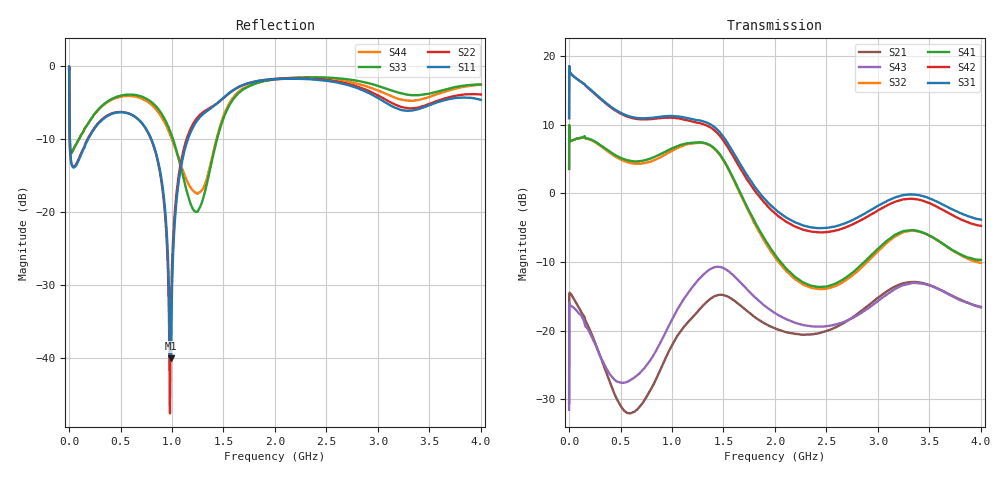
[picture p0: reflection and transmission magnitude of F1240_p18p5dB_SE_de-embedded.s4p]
! Integrated Device Technology
! Corporate Headquarters
! 6024 Silver Creek Valley Road
! San Jose, CA 95138  USA
! Phone:  1-408-284-8200
! Toll Free:  1-800-223-1366
! Webpage:  http://www.idt.com/
! Timing and RF Division
! 515 Groton Road, Suite 102
! Westford, MA 01886-6024
! Device:  F1240
! Description: Dual Intermediate Frequency Digital Variable Gain Amplifier
! Frequency:  10.0 -  500.00 MHz
! Package:  5x5 mm QFN Plastic Package: 32 pin
! Ports:  8 RF, 20 DC
!  Pin  1  = GA3 / Data  Pin 17  = RF OUT_B+
!  Pin  2  = GA4 / CLK  Pin 18  = RF OUT_B-
!  Pin  3  = GA5  Pin 19  = STBY_B
!  Pin  4  = VMODE  Pin 20  = Ground
!  Pin  5  = No Connect  Pin 21  = Ground
!  Pin  6  = GB5  Pin 22  = STB_A
!  Pin  7  = GB4  Pin 23  = RF OUT_A-  = Port 4
!  Pin  8  = GB3  Pin 24  = RF OUT_A+  = Port 3
!  Pin  9  = GB2  Pin 25  = GA0
!  Pin 10  = GB1  Pin 26  = ISET_A
!  Pin 11  = RF IN_B+  Pin 27  = VCC
!  Pin 12  = RF IN_B-  Pin 28  = Ground
!  Pin 13  = Ground  Pin 29  = RF IN_A-  = Port 2
!  Pin 14  = VCC  Pin 30  = RF IN_A+  = Port 1
!  Pin 15  = ISET_B  Pin 31  = GA1
!  Pin 16  = GB0  Pin 32  = GA2 / CSb
! Gain  = +19.5 dB
! State  = 1
! Voltage  = +5.00 V
! Current  = 85.292 mA (one channel only)
! Temperture  =  +25 C
! Test Date  =  2017-10-18
! Board  =  EB4031
! Data:  The device was measured on a custom evaluation board which has
!  individual transmission lines to the RF pins.  Data was collected
!  using a calibrated network analyzer.  The evaluation board was
!  de-embedded using Automatic Fixture Removal.
!  The reference plane is the edge of the package pin.
!  Only Channel A was measured.
!  This data is in single-ended operation.  If your needs are balanced
!  or differential S-parameters then this file needs to be used a
!  linear simulator.
! File Date:  2017-11-10  MJV
! Note:
!  Integrated Device Technology supplies this data as a sample of measured
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# Hz S dB R 100
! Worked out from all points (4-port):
!   410 points, 500 kHz to 4 GHz, reference 100 ohm
!   strongest paths, dB at 500 kHz, 930 MHz, 1.96 GHz, 2.98 GHz, 4 GHz:
!     S31: 11.0, 11.2, -1.8, -2.0, -3.8
!     S42: 10.9, 11.0, -2.4, -2.7, -4.7
!     S41: 3.5, 6.0, -8.1, -8.4, -9.7
!     S32: 3.5, 5.6, -8.5, -8.8, -10.1
!     S43: -31.5, -20.5, -17.1, -15.9, -16.5
!     S21: -30.6, -24.3, -19.4, -15.5, -16.6
!   lowest |S11| = -40.0 dB at 990 MHz (marker M1), VSWR 1.02, Z = 101 - j1.89 ohm
!   |S11| at or under -10 dB: 7.315 MHz to 183.5 MHz (176.2 MHz wide, 185 % of centre); 800.1 MHz to 1.153 GHz (353.1 MHz wide, 36.2 % of centre)
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500000  -0.28 -6.7  -30.39 27.2  -27.54 71.4  -64.34 71.3
        -30.57 26.5  -0.27 -6.6  -63.97 65.9  -27.55 72.5
        10.95 -105.6  3.54 72.6  -0.39 0.6  -31.58 -174.7
        3.54 73.6  10.93 -104.4  -31.54 -174.8  -0.40 3.0
3500000  -6.39 -49.9  -14.55 14.8  -21.30 7.1  -38.64 42.3
         -14.56 14.7  -6.36 -50.0  -38.60 42.2  -21.31 7.2
         18.14 -171.8  8.30 -1.1  -6.05 -44.7  -16.10 25.3
         8.29 -1.1  18.13 -171.6  -16.07 25.2  -6.10 -44.5
2.1e8  -9.33 -110.6  -20.17 -111.1  -24.08 -52.3  -33.44 7.8
       -20.20 -109.9  -9.19 -112.4  -33.46 7.8  -24.10 -52.2
       15.10 106.5  7.76 -61.4  -7.26 -79.5  -20.09 -118.6
       7.85 -61.3  15.03 105.6  -20.62 -117.2  -7.29 -78.8
5.6e8  -6.38 -172.2  -31.15 93.4  -25.65 -107.5  -27.51 -61.3
       -31.98 91.5  -6.35 -173.6  -27.68 -60.1  -25.82 -107.8
       11.33 19.8  4.55 -146.2  -3.87 -151.4  -26.39 91.3
       4.83 -147.1  11.20 18.7  -27.50 68.5  -4.04 -150.8
9.9e8  -39.99 -70.0  -20.56 -32.2  -22.54 164.1  -22.61 -162.8
       -22.43 -32.5  -32.93 -58.3  -22.97 -158.5  -22.98 163.6
       11.26 -83.9  6.10 120.9  -9.19 146.8  -17.37 -11.3
       6.47 115.9  11.01 -85.7  -18.69 -34.2  -9.63 153.2
1.5e9  -4.28 -138.4  -14.87 166.6  -29.55 43.3  -24.07 69.5
       -14.84 171.9  -4.33 -139.7  -24.10 75.5  -31.33 37.8
       8.19 119.0  4.78 -56.1  -7.10 -112.2  -10.52 165.6
       4.86 -61.1  7.66 117.4  -10.89 158.2  -6.75 -115.9
4e9  -4.56 -158.7  -16.66 54.1  -22.00 -34.3  -19.29 -48.2
     -16.62 53.5  -3.84 -152.0  -21.87 -29.5  -25.70 -15.1
     -3.84 -3.8  -10.14 -145.0  -2.48 -135.7  -14.60 89.3
     -9.71 -155.0  -4.74 5.0  -16.55 63.0  -2.49 -140.5
